|Texas Instruments Incorporated
| Put part description here: 1000Base-T1 Automotive Ethernet
| Marketing Part # : DP83TG720
| Digital Voltage Range : 1V
| Package-type: 36 QFN
| #pins/pkg drawing : 36-pin QFN
[IBIS Ver] 4.1
[File name] dp83tg720s.ibs
[File Rev] 2.2
[Date] 08/14/2020
[Source]
| Texas Instruments Incorporated.
| 12500 TI Blvd
| Dallas, TX -75243
[Notes] Revision History:
| Rev 2.2: Updated version with corrected typo in pin names
| Rev 2.1: Updated pin mapping on led_0 and led_1
| Rev 1.0: 07/15/2020
| - Initial version of the model
| - Model generated from simulations in TISPICE/SPECTRE
| - C_comp although listed in numerical order of value are
| obtained from varying PVT conditions. For PVT conditions for
| each specific value refer the buffer description under
| respective [Model]. IBIS model user is responsible for using
| appropriate C_comp to simulate for Signal Integrity.
| - Warnings regarding combined Non-monotonicity of various models have been
| reviewed and considered minor and can be ignored.
|**** Modify the following if you use [Model Selector]*****************
| - Model names with a trailing _1p8 contain the model for
| 1.8V operation. Model names with a trailing _3p3 contain the model
| for 3.3V operation.
[Disclaimer]
| This model is designed as an aid for customers of Texas Instruments.
| TI and its licensors and suppliers make no warranties, either expressed
| or implied, with respect to this model, including the warranties of
| merchantability or fitness for a particular purpose. The model is
| provided solely on an "as is" basis. The entire risk as to its quality
| and performance is with the customer.
| This model is subject to change without notice. Texas Instruments
| Incorporated is not responsible for updating this model.
[Copyright]
(C) Copyright 2019 Texas Instruments Incorporated. All rights reserved.
| Component1 DP83TG720
[Component] DP83TG720
[Manufacturer]	Texas Instruments Incorporated
[Package] 	|36 QFN Wettable Flank Package
| variable typ min max
R_pkg 0.05 0.04 0.06
L_pkg 1.0nH 0.8nH 1.2nH
C_pkg 0.2pF 0.16pF 0.24pF
| pin number (pin name) mapping to model name
[Pin] signal_name model_name R_pin L_pin C_pin
1   MDC   gpio_rgmii_mtx_grx_mdc_mdio   0.1 1.2nH   0.2pF
2   INT_N   gpio_rgmii_mtx_grx_od   0.1 1.2nH   0.2pF
3   RESET_N   gpio_rgmii_mtx_grx_od   0.1 1.2nH   0.2pF
4   XO   NC   0.1 1.2nH   0.2pF
5   XI   NC   0.1 1.2nH   0.2pF
6   LED_1   gpio_rgmii_gtx_mrx   0.1 1.2nH   0.2pF
7   VSLEEP   POWER   0.1 1.2nH   0.2pF
8   WAKE   input_buffer_wake_vsleep   0.1 1.2nH   0.2pF
9   VDD1P0   POWER   0.1 1.2nH   0.2pF
10   INH   gpo_inh   0.1 1.2nH   0.2pF
11   VDDA3P3   POWER   0.1 1.2nH   0.2pF
12   TRD_P   NC   0.1 1.2nH   0.2pF
13   TRD_M   NC   0.1 1.2nH   0.2pF
14   STRP_1   gpio_rgmii_gtx_mrx_4levelstrap   0.1 1.2nH   0.2pF
15   RX_CTRL   gpio_rgmii_gtx_mrx_4levelstrap   0.1 1.2nH   0.2pF
16   CLKOUT   gpio_rgmii_gtx_mrx_clkout   0.1 1.2nH   0.2pF
17   DNC   NC   0.1 1.2nH   0.2pF
18   DNC   input_buffer   0.1 1.2nH   0.2pF
19   DNC   NC   0.1 1.2nH   0.2pF
20   DNC   NC   0.1 1.2nH   0.2pF
21   VDD1P0   POWER   0.1 1.2nH   0.2pF
22   VDDIO   POWER   0.1 1.2nH   0.2pF
23   RX_D3   sgmii_tx   0.1 1.2nH   0.2pF
24   RX_D2   sgmii_tx   0.1 1.2nH   0.2pF
25   RX_D1   gpio_rgmii_gtx_mrx   0.1 1.2nH   0.2pF
26   RX_D0   gpio_rgmii_gtx_mrx   0.1 1.2nH   0.2pF
27   RX_CLK   gpio_rgmii_gtx_mrx   0.1 1.2nH   0.2pF
28   TX_CLK   gpio_rgmii_mtx_grx   0.1 1.2nH   0.2pF
29   TX_CTRL   gpio_rgmii_mtx_grx   0.1 1.2nH   0.2pF
30   TX_D3   gpio_rgmii_mtx_grx   0.1 1.2nH   0.2pF
31   TX_D2   gpio_rgmii_mtx_grx   0.1 1.2nH   0.2pF
32   TX_D1   sgmii_rx   0.1 1.2nH   0.2pF
33   TX_D0   sgmii_rx   0.1 1.2nH   0.2pF
34   VDDIO   POWER   0.1 1.2nH   0.2pF
35   LED_0   gpio_rgmii_gtx_mrx   0.1 1.2nH   0.2pF
36   MDIO   gpio_rgmii_mtx_grx_mdc_mdio   0.1 1.2nH   0.2pF
| Use Differential pin definition for differential I/Os (If Differential pin pairs are modeled)
[Diff Pin] inv_pin vdiff tdelay_typ tdelay_min tdelay_max
24 23 100mV NA NA NA
32 33 100mV NA NA NA
|***** end of component 1 definition
| Model Selectors
|For RGMII RX lines and clkout, mode00=default IO slew; mode10=fast IO slew; mode01= slow IO slew;
|NOTE: The default register settings on-chip for RGMII RX lines is mode10.
|NOTE: The default register settings on-chip for clkout is mode00
[Model Selector] gpio_rgmii_gtx_mrx
ibis_gtx_mrx_mode10_1p8 at VDDIO 1.8V operation.
ibis_gtx_mrx_mode10_2p5v at 2.5V operation.
ibis_gtx_mrx_mode10_3p3v at 3.3V operation.
ibis_gtx_mrx_mode01_1p8v at 1.8V operation.
ibis_gtx_mrx_mode01_2p5v at 2.5V operation.
ibis_gtx_mrx_mode01_3p3v at 3.3V operation.
ibis_gtx_mrx_mode00_1p8v at 1.8V operation.
ibis_gtx_mrx_mode00_2p5v at 2.5V operation.
ibis_gtx_mrx_mode00_3p3v at 3.3V operation.
[Model Selector] gpio_rgmii_gtx_mrx_sgmii_off
ibis_sgmii_off_gtx_mrx_mode10_1p8 at VDDIO 1.8V operation.
ibis_sgmii_off_gtx_mrx_mode10_2p5v at VDDIO 2.5V operation.
ibis_sgmii_off_gtx_mrx_mode10_3p3v at VDDIO 3.3V operation.
ibis_sgmii_off_gtx_mrx_mode01_1p8v at VDDIO 1.8V operation.
ibis_sgmii_off_gtx_mrx_mode01_2p5v at VDDIO 2.5V operation.
ibis_sgmii_off_gtx_mrx_mode01_3p3v at VDDIO 3.3V operation.
ibis_sgmii_off_gtx_mrx_mode00_1p8v at VDDIO 1.8V operation.
ibis_sgmii_off_gtx_mrx_mode00_2p5v at VDDIO 2.5V operation.
ibis_sgmii_off_gtx_mrx_mode00_3p3v at VDDIO 3.3V operation.
[Model Selector] gpio_rgmii_gtx_mrx_4levelstrap
ibis_gtx_mrx_4levelstraps_mode10_1p8 at VDDIO 1.8V operation.
ibis_gtx_mrx_4levelstraps_mode10_2p5v at VDDIO 2.5V operation.
ibis_gtx_mrx_4levelstraps_mode10_3p3v at VDDIO 3.3V operation.
ibis_gtx_mrx_4levelstraps_mode01_1p8v at VDDIO 1.8V operation.
ibis_gtx_mrx_4levelstraps_mode01_2p5v at VDDIO 2.5V operation.
ibis_gtx_mrx_4levelstraps_mode01_3p3v at VDDIO 3.3V operation.
ibis_gtx_mrx_4levelstraps_mode00_1p8v at VDDIO 1.8V operation.
ibis_gtx_mrx_4levelstraps_mode00_2p5v at VDDIO 2.5V operation.
ibis_gtx_mrx_4levelstraps_mode00_3p3v at VDDIO 3.3V operation.
[Model Selector] gpio_rgmii_mtx_grx
gpio_mtx_grx_1p8v_pupd10 at VDDIO 1.8V operation.
gpio_mtx_grx_2p5v_pupd10 at VDDIO 2.5V operation.
gpio_mtx_grx_3p3v_pupd10 at VDDIO 3.3V operation.
[Model Selector] gpio_rgmii_mtx_grx_sgmii_off
ibis_sgmii_off_mtx_grx_1p8 at VDDIO 1.8V operation.
ibis_sgmii_off_mtx_grx_2p5 at VDDIO 2.5V operation.
ibis_sgmii_off_mtx_grx_3p3 at VDDIO 3.3V operation.
[Model Selector] gpio_rgmii_gtx_mrx_clkout
ibis_clkout_gtx_mrx_mode01_1p8v at VDDIO 1.8V operation.
ibis_clkout_gtx_mrx_mode10_1p8v at VDDIO 1.8V operation.
ibis_clkout_gtx_mrx_mode10_2p5v at VDDIO 2.5V operation.
ibis_clkout_gtx_mrx_mode10_3p3v at VDDIO 3.3V operation.
ibis_clkout_gtx_mrx_mode01_2p5v at VDDIO 2.5V operation.
ibis_clkout_gtx_mrx_mode01_3p3v at VDDIO 3.3V operation.
ibis_clkout_gtx_mrx_mode00_1p8v at VDDIO 1.8V operation.
ibis_clkout_gtx_mrx_mode00_2p5v at VDDIO 2.5V operation.
ibis_clkout_gtx_mrx_mode00_3p3v at VDDIO 3.3V operation.
[Model Selector] input_buffer
input_buffer_1p8v at VDDIO 1.8V operation
input_buffer_2p5v at VDDIO 2.5V operation
input_buffer_3p3v at VDDIO 3.3V operation
[Model Selector] input_buffer_wake_vsleep
input_buffer_wake at VSLEEP 3.3V operation.
[Model Selector] gpio_rgmii_mtx_grx_od
gpio_mtx_grx_1p8v_pupd01 at VDDIO 1.8V operation.
gpio_mtx_grx_2p5v_pupd01 at VDDIO 2.5V operation.
gpio_mtx_grx_3p3v_pupd01 at VDDIO 3.3V operation.
[Model Selector] gpo_inh
ibis_gpo_inh_3p3v at 3.3V operation
[Model Selector] gpio_rgmii_mtx_grx_mdc_mdio
gpio_mtx_grx_1p8v_pupd00 at VDDIO 1.8V operation.
gpio_mtx_grx_2p5v_pupd00 at VDDIO 2.5V operation.
gpio_mtx_grx_3p3v_pupd00 at VDDIO 3.3V operation.
[Model Selector] sgmii_tx
ibis_sgmii_tx at SGMII 3.3V operation.
[Model Selector] sgmii_rx
ibis_sgmii_rx at SGMII 3.3V operation.
| Models and submodels in the file (55): ibis_gtx_mrx_mode10_1p8 (I/O), ibis_sgmii_off_gtx_mrx_mode10_1p8 (I/O), ibis_gtx_mrx_4levelstraps_mode10_1p8 (I/O), gpio_mtx_grx_1p8v_pupd10 (I/O), ibis_sgmii_off_mtx_grx_1p8 (I/O), gpio_mtx_grx_1p8v_pupd00 (I/O), ibis_clkout_gtx_mrx_mode01_1p8v (I/O), ibis_gtx_mrx_mode10_2p5v (I/O), ibis_gtx_mrx_mode10_3p3v (I/O), ibis_gtx_mrx_mode01_1p8v (I/O), ibis_gtx_mrx_mode01_2p5v (I/O), ibis_gtx_mrx_mode01_3p3v (I/O), ibis_gtx_mrx_mode00_1p8v (I/O), ibis_gtx_mrx_mode00_2p5v (I/O), ibis_gtx_mrx_mode00_3p3v (I/O), ibis_sgmii_off_gtx_mrx_mode10_2p5v (I/O), ibis_sgmii_off_gtx_mrx_mode10_3p3v (I/O), ibis_sgmii_off_gtx_mrx_mode01_1p8v (I/O), ibis_sgmii_off_gtx_mrx_mode01_2p5v (I/O), ibis_sgmii_off_gtx_mrx_mode01_3p3v (I/O), ibis_sgmii_off_gtx_mrx_mode00_1p8v (I/O), ibis_sgmii_off_gtx_mrx_mode00_2p5v (I/O), ibis_sgmii_off_gtx_mrx_mode00_3p3v (I/O), ibis_clkout_gtx_mrx_mode10_1p8v (I/O), ibis_clkout_gtx_mrx_mode10_2p5v (I/O), ibis_clkout_gtx_mrx_mode10_3p3v (I/O), ibis_clkout_gtx_mrx_mode01_2p5v (I/O), ibis_clkout_gtx_mrx_mode01_3p3v (I/O), ibis_clkout_gtx_mrx_mode00_1p8v (I/O), ibis_clkout_gtx_mrx_mode00_2p5v (I/O), ibis_clkout_gtx_mrx_mode00_3p3v (I/O), ibis_gtx_mrx_4levelstraps_mode10_2p5v (I/O), ibis_gtx_mrx_4levelstraps_mode10_3p3v (I/O), ibis_gtx_mrx_4levelstraps_mode01_1p8v (I/O), ibis_gtx_mrx_4levelstraps_mode01_2p5v (I/O), ibis_gtx_mrx_4levelstraps_mode01_3p3v (I/O), ibis_gtx_mrx_4levelstraps_mode00_1p8v (I/O), ibis_gtx_mrx_4levelstraps_mode00_2p5v (I/O), ibis_gtx_mrx_4levelstraps_mode00_3p3v (I/O), gpio_mtx_grx_2p5v_pupd10 (I/O), gpio_mtx_grx_3p3v_pupd10 (I/O), gpio_mtx_grx_2p5v_pupd00 (I/O), gpio_mtx_grx_3p3v_pupd00 (I/O), gpio_mtx_grx_1p8v_pupd01 (I/O), gpio_mtx_grx_2p5v_pupd01 (I/O), gpio_mtx_grx_3p3v_pupd01 (I/O), input_buffer_wake (Input), input_buffer_1p8v (Input), input_buffer_2p5v (Input), input_buffer_3p3v (Input), ibis_sgmii_off_mtx_grx_2p5 (Input), ibis_sgmii_off_mtx_grx_3p3 (Input), ibis_gpo_inh_3p3v (Open_source), ibis_sgmii_tx (Output), ibis_sgmii_rx (Input)
